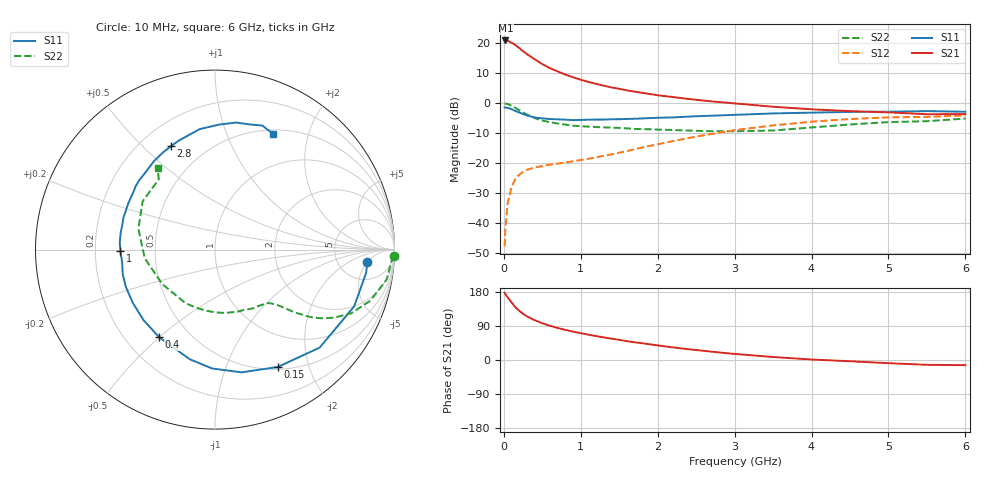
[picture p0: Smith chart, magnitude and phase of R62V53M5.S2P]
! SIEMENS Small Signal Semiconductors
! BFR193
! Si NPN RF Bipolar Junction Transistor in SOT23
! VCE = 2.5 V  IC = 3.5 mA
! Common Emitter S-Parameters:  May  1996
# GHz  S  MA  R  50
!  f  S11  S21  S12  S22
! GHz  MAG  ANG  MAG  ANG  MAG  ANG  MAG  ANG
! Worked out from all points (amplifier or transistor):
!   36 points, 10 MHz to 6 GHz, reference 50 ohm
!   highest |S21| = 21.0 dB at 20 MHz (marker M1)
!   |S21| within 3 dB of that: start of sweep to 222.9 MHz
!   unconditionally stable (mu >= 1): 990.5 MHz to 2.029 GHz
!   at 250 MHz: K = 0.34, MSG = 20.2 dB, |S12| = -22.9 dB
!   at 1.4 GHz: K = 1.08, MAG = 9.4 dB, |S12| = -17.1 dB
!   at 6 GHz: K = 0.98, MSG = 0.2 dB, |S12| = -4.1 dB
!   S11 on the Smith chart (normalised r, x): 10 MHz: 10, -5; 150 MHz: 0.53, -1.54; 400 MHz: 0.34, -0.50; 1 GHz: 0.31, -0.01; 2.8 GHz: 0.32, +0.61; 6 GHz: 0.55, +1.47
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0.01  0.8516 -4.5  11.09 177.3  0.0041 90.4  0.9955 -2.0
0.02  0.8519 -8.8  11.2 173.9  0.0084 87.0  0.9849 -3.9
0.05  0.8374 -22.2  11.11 165.2  0.0215 78.7  0.9714 -9.8
0.1  0.7988 -43.1  10.27 152.0  0.0396 68.6  0.911 -18.2
0.15  0.7418 -61.8  9.387 139.3  0.0543 60.0  0.8383 -25.0
0.2  0.6999 -77.7  8.406 129.8  0.0641 53.8  0.764 -29.8
0.25  0.6626 -91.4  7.405 121.8  0.0715 49.0  0.7005 -33.1
0.3  0.6271 -102.9  6.644 115.2  0.0774 46.1  0.6502 -35.3
0.4  0.579 -122.4  5.456 105.2  0.0845 42.8  0.5666 -38.2
0.5  0.5595 -135.4  4.503 97.0  0.0892 41.5  0.5135 -39.8
0.6  0.5457 -147.0  3.862 90.4  0.0943 41.5  0.4826 -40.8
0.7  0.5385 -157.2  3.402 84.5  0.0981 42.3  0.4591 -42.0
0.8  0.5324 -164.9  3.017 79.5  0.1026 43.5  0.4397 -43.3
1  0.5268 -179.0  2.473 70.8  0.1126 47.8  0.4144 -46.4
1.1  0.5322 175.8  2.274 66.8  0.1185 49.8  0.4068 -48.6
1.6  0.5472 152.3  1.642 49.7  0.159 57.1  0.3809 -60.8
2.2  0.5806 131.2  1.269 33.2  0.2337 58.5  0.3574 -81.0
2.8  0.6265 113.0  1.048 19.9  0.3234 53.2  0.3401 -108.2
3.5  0.6767 97.2  0.875 7.9  0.4268 41.9  0.351 -146.8
4.5  0.7176 80.6  0.739 -3.3  0.5457 23.6  0.4423 164.8
5.5  0.7396 69.1  0.656 -12.7  0.5912 5.7  0.5018 128.6
6  0.722 63.5  0.66 -13.7  0.6268 0.7  0.5563 125.1
